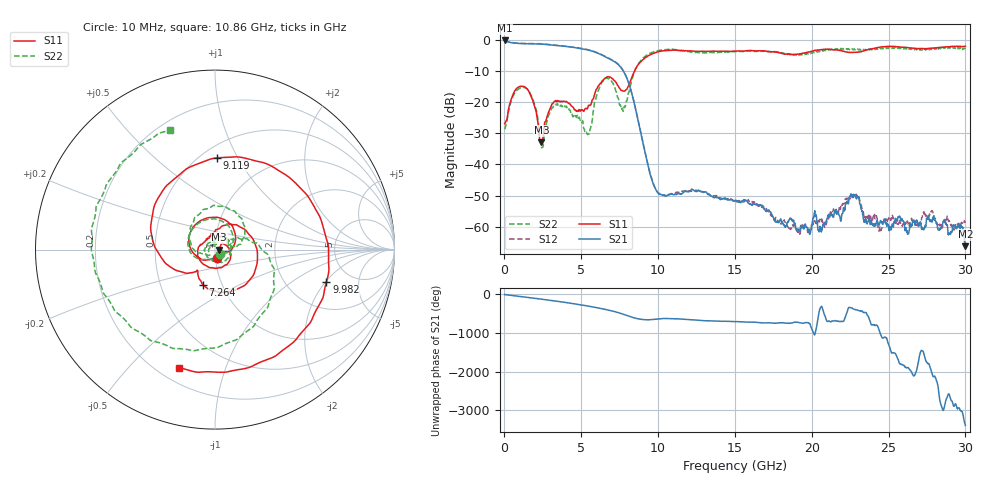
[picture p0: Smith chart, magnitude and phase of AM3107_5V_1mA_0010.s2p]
# Hz S DB R 50.0
!freq dBS11 angS11 dBS21 angS21 dBS12 angS12 dBS22 angS22
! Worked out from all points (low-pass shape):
!   1601 points, 10 MHz to 30 GHz, reference 50 ohm
!   highest |S21| = -0.09 dB at 10 MHz (marker M1); lowest = -66.3 dB at 30 GHz (marker M2)
!   |S21| within 3 dB of the highest: start of sweep to 5.381 GHz
!   lowest |S11| = -32.9 dB at 2.409 GHz (marker M3), VSWR 1.05, Z = 52.3 + j0.0258 ohm
!   |S11| at or under -10 dB: start of sweep to 8.461 GHz
!   |S22| runs from -34.6 to -2.2 dB; largest |S21 - S12| = 0.012
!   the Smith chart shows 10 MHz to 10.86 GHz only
!   S11 on the Smith chart (normalised r, x): 10 MHz: 1.02, -0.09; 7.264 GHz: 0.81, -0.34; 9.119 GHz: 0.60, +0.83; 9.982 GHz: 3.29, -2.05; 10.86 GHz: 0.28, -0.70
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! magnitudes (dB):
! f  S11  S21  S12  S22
! 10 MHz  -26.9  -0.1  -0.1  -28.7
! 609.8 MHz  -16.9  -0.9  -0.8  -17.5
! 1.341 GHz  -15.1  -1.1  -1.1  -15.3
! 1.959 GHz  -21.2  -1.2  -1.1  -20.6
! 2.409 GHz  -32.9  -1.2  -1.2  -34.4
! 3.309 GHz  -19.5  -1.7  -1.6  -20.7
! 5.015 GHz  -22.4  -2.7  -2.6  -26.2
! 5.521 GHz  -21.0  -3.3  -3.2  -30.1
! 6.477 GHz  -12.5  -5.1  -5.0  -12.7
! 7.264 GHz  -13.6  -7.2  -7.1  -16.5
! 7.751 GHz  -16.4  -10.0  -9.9  -22.6
! 9.119 GHz  -5.8  -35.5  -35.4  -5.3
! 9.982 GHz  -3.8  -49.1  -49.0  -3.4
! 10.02 GHz  -3.7  -49.3  -49.3  -3.4
! 10.86 GHz  -3.3  -49.4  -49.5  -3.0
! 15.01 GHz  -3.5  -51.8  -51.8  -3.6
! 20.01 GHz  -3.6  -59.9  -59.4  -4.2
! 22.67 GHz  -3.9  -49.9  -50.1  -3.0
! 24.45 GHz  -2.2  -58.3  -60.1  -2.6
! 25.01 GHz  -2.0  -61.1  -57.4  -2.6
! 27.92 GHz  -2.6  -56.8  -56.4  -2.8
! 30 GHz  -1.9  -66.3  -58.5  -2.4
